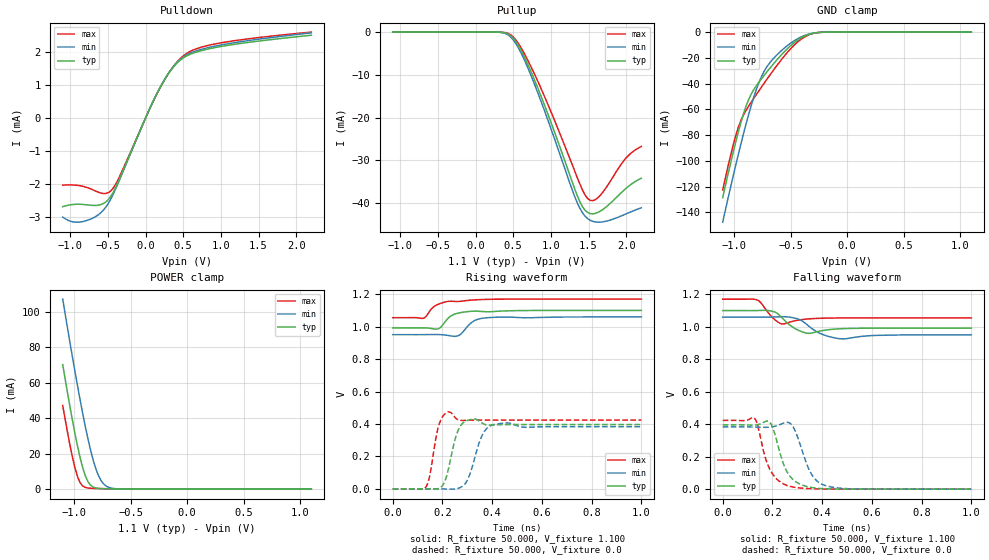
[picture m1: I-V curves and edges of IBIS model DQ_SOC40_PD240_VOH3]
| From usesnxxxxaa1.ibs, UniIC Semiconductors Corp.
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|   Model DQ_SOC40_PD240_VOH3
[Model] DQ_SOC40_PD240_VOH3
Model_type I/O
Polarity   Non-Inverting
Enable   Active-High
Vinl =  0.113V
Vinh =  0.253V
Vmeas =  0.183V
Rref =  50.000
Vref =  0.183V
C_comp   1.110pF   1.087pF   1.118pF
[Model Spec]
Vinh   0.253V   0.247V   0.265V
Vinl   0.113V   0.107V   0.125V
Vmeas   0.183V   NA   NA
Vref   0.183V   NA   NA
Rref   50.000   NA   NA
[Temperature Range]   25.000   0.125k   -40.000
[Voltage Range]   1.100V   1.060V   1.170V
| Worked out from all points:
|   slope of the pulldown table from 0 to 0.165 V, typ, clamps not added: 206 ohm
|   GND clamp passes 1 mA (typ) near -0.30 V on its own axis
|   POWER clamp passes 1 mA (typ) near -0.82 V on its own axis
|   rising waveform, R_fixture 50.000, V_fixture 1.100: 20-80 % time 49ps typ, 44.8ps min, 58.7ps max; typ from 0.992 V to 1.1 V
|   rising waveform, R_fixture 50.000, V_fixture 0.0: 20-80 % time 36ps typ, 46.7ps min, 27.4ps max; typ from 0 V to 0.396 V
|   falling waveform, R_fixture 50.000, V_fixture 1.100: 20-80 % time 44.8ps typ, 58.3ps min, 34ps max; typ from 1.1 V to 0.992 V
|   falling waveform, R_fixture 50.000, V_fixture 0.0: 20-80 % time 56.7ps typ, 59.3ps min, 55.8ps max; typ from 0.396 V to 0 V
[Pulldown]
|Voltage   I(typ)   I(min)   I(max)
-1.1V     -2.687mA   -3.002mA   -2.035mA
-930mV    -2.614mA   -3.157mA   -2.036mA
-726mV    -2.644mA   -3.06mA    -2.15mA
-556mV    -2.587mA   -2.78mA    -2.289mA
-454mV    -2.347mA   -2.422mA   -2.193mA
-352mV    -1.879mA   -1.911mA   -1.806mA
158mV     771.5uA    774.7uA    764.3uA
328mV     1.42mA     1.434mA    1.431mA
498mV     1.814mA    1.841mA    1.876mA
668mV     1.992mA    2.028mA    2.091mA
974mV     2.154mA    2.199mA    2.264mA
2.2V      2.506mA    2.578mA    2.601mA
[Pullup]
|Voltage   I(typ)   I(min)   I(max)
-1.1V     1nA        40.29nA    -1.059nA
432mV     -445.9uA   -664.3uA   -301.9uA
568mV     -3.14mA    -3.672mA   -2.666mA
738mV     -9.312mA   -10.23mA   -8.171mA
976mV     -19.93mA   -21.36mA   -17.58mA
1.316V    -36.64mA   -38.44mA   -32.48mA
1.418V    -40.78mA   -42.2mA    -36.86mA
1.486V    -42.14mA   -43.56mA   -38.87mA
1.554V    -42.47mA   -44.22mA   -39.39mA
1.622V    -42.15mA   -44.42mA   -38.73mA
1.996V    -36.53mA   -42.49mA   -29.45mA
2.2V      -34.15mA   -41.04mA   -26.73mA
[GND_clamp]
|Voltage   I(typ)   I(min)   I(max)
-1.1V     -128.5mA   -147.6mA   -122.6mA
-1.008V   -93.62mA   -112mA     -87.95mA
-962mV    -77.6mA    -95.05mA   -73.96mA
-893mV    -57.36mA   -71.21mA   -60.7mA
-847mV    -48.01mA   -56.81mA   -54.36mA
-801mV    -41.47mA   -44.23mA   -48.33mA
-755mV    -36.02mA   -34.19mA   -42.41mA
-709mV    -30.9mA    -26.94mA   -36.63mA
-525mV    -12.67mA   -10.3mA    -15.49mA
-387mV    -3.615mA   -3.065mA   -4.419mA
-249mV    -281uA     -330.6uA   -301.3uA
1.1V      0A         0A         0A
[POWER_clamp]
|Voltage   I(typ)   I(min)   I(max)
-1.1V     70.27mA    107.3mA    47.25mA
-1.039V   47.68mA    83.93mA    25.86mA
-993mV    31.88mA    66.94mA    12.35mA
-970mV    24.65mA    58.72mA    7.262mA
-947mV    18.06mA    50.74mA    3.761mA
-901mV    7.73mA     35.71mA    987.1uA
-855mV    2.348mA    22.46mA    514uA
-809mV    697.3uA    11.94mA    396.5uA
-763mV    321uA      5.097mA    322.7uA
-717mV    213.8uA    1.813mA    258.1uA
-556mV    65.24uA    79.15uA    81.64uA
1.1V      0A         0A         0A
[Ramp]
| variable   typ   min   max
dV/dt_r   0.238/36.627p   0.230/46.763p   0.254/27.667p
dV/dt_f   64.848m/44.917p   65.673m/58.755p   68.888m/34.127p
R_load = 50.000
[Rising Waveform]
R_fixture= 50.000
V_fixture= 1.100
V_fixture_min= 1.060
V_fixture_max= 1.170
|time   V(typ)   V(min)   V(max)
0s        991.9mV    950.6mV    1.055V
122ps     992.6mV    950.6mV    1.051V
134ps     992.1mV    950.8mV    1.063V
163ps     986.7mV    951.3mV    1.12V
181ps     985.6mV    951.2mV    1.137V
225ps     1.054V     945.2mV    1.156V
262ps     1.083V     942.8mV    1.155V
319ps     1.095V     1.028V     1.164V
379ps     1.092V     1.055V     1.168V
1ns       1.1V       1.06V      1.17V
[Rising Waveform]
R_fixture= 50.000
V_fixture= 0.0
V_fixture_min= 0.0
V_fixture_max= 0.0
|time   V(typ)   V(min)   V(max)
0s        3.61uV     29.2uV     671nV
135ps     -17.94uV   102uV      13.82mV
184ps     2.406mV    95.49uV    385.2mV
223ps     115.7mV    -1.636mV   474.5mV
252ps     311.9mV    -934.7uV   437.5mV
282ps     405.6mV    17.2mV     421.4mV
312ps     426.9mV    95.77mV    423.1mV
358ps     407.1mV    323.9mV    423.7mV
398ps     392.5mV    392.1mV    423.7mV
1ns       396.3mV    383.1mV    423.7mV
[Falling Waveform]
R_fixture= 50.000
V_fixture= 1.100
V_fixture_min= 1.060
V_fixture_max= 1.170
|time   V(typ)   V(min)   V(max)
0s        1.1V       1.06V      1.17V
140ps     1.1V       1.06V      1.165V
202ps     1.095V     1.061V     1.055V
238ps     1.057V     1.062V     1.018V
283ps     996.8mV    1.056V     1.034V
333ps     962.5mV    1.021V     1.047V
390ps     973.5mV    960.4mV    1.052V
470ps     987.7mV    926.7mV    1.055V
618ps     991.7mV    947.3mV    1.055V
1ns       991.9mV    950.5mV    1.055V
[Falling Waveform]
R_fixture= 50.000
V_fixture= 0.0
V_fixture_min= 0.0
V_fixture_max= 0.0
|time   V(typ)   V(min)   V(max)
0s        396.3mV    383.1mV    423.7mV
127ps     394.6mV    382.7mV    438.6mV
184ps     418.1mV    381.5mV    141.2mV
202ps     376mV      384.6mV    90.78mV
237ps     188.5mV    402.1mV    38.72mV
265ps     90.61mV    410.2mV    19.47mV
293ps     46.69mV    354mV      10.63mV
359ps     10.04mV    87.03mV    2.698mV
409ps     2.886mV    24.1mV     947.3uV
1ns       7.401uV    32.4uV     -7.388uV
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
